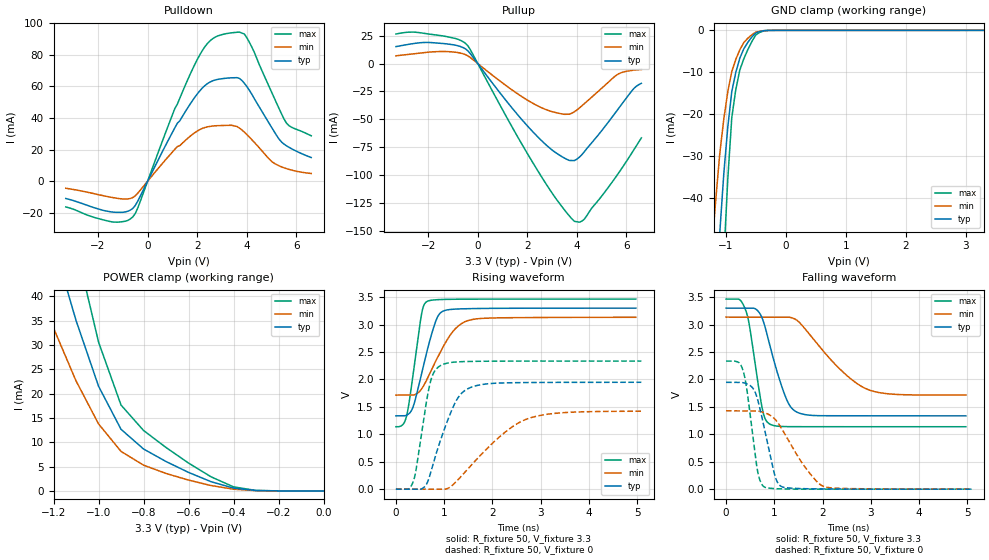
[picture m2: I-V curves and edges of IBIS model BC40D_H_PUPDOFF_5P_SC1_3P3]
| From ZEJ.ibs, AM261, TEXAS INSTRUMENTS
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[Model]   BC40D_H_PUPDOFF_5P_SC1_3P3
Model_type   I/O
Polarity   Non-Inverting
Enable   Active-Low
Vinl =  0.8V
Vinh =  2V
Cref =  15pF
Rref =  100.0000M
Vref =  0V
Vmeas =  1.65
C_comp   2.157014p   1.964007p   2.198404p
|[Input load] weak_pupdoff
|[Output drive] slow
|[supplytol] 5
|[temp] ind
[Model Spec]
Vinl   0.8V   0.8V   0.8V
Vinh   2V   2V   2V
[Temperature Range]   25   125   -40
[Voltage Range]   3.3   3.135   3.465
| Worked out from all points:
|   slope of the pulldown table from 0 to 0.495 V, typ, clamps not added: 31.8 ohm
|   slope of the pullup table from 0 to 0.495 V, typ, clamps not added: 33.8 ohm
|   GND clamp passes 1 mA (typ) near -0.53 V on its own axis
|   POWER clamp passes 1 mA (typ) near -0.43 V on its own axis
|   rising waveform, R_fixture 50, V_fixture 3.3: 20-80 % time 338ps typ, 517ps min, 220ps max; typ from 1.34 V to 3.3 V
|   rising waveform, R_fixture 50, V_fixture 0: 20-80 % time 469ps typ, 1.01ns min, 254ps max; typ from 0 V to 1.95 V
|   falling waveform, R_fixture 50, V_fixture 3.3: 20-80 % time 389ps typ, 896ps min, 241ps max; typ from 3.3 V to 1.34 V
|   falling waveform, R_fixture 50, V_fixture 0: 20-80 % time 295ps typ, 611ps min, 205ps max; typ from 1.95 V to 0 V
| Nom Voltages:
|   VDD=1.1, VDDS=3.3, VDDS18=1.8, ESD_BIASFET=0, VSS=0, VSSS=0
| Min Voltages:
|   VDD=1.045, VDDS=3.135, VDDS18=1.71, ESD_BIASFET=0, VSS=0, VSSS=0
| Max Voltages:
|   VDD=1.16, VDDS=3.465, VDDS18=1.89, ESD_BIASFET=0, VSS=0, VSSS=0
[POWER_clamp]
|   voltage   I(typ)   I(min)   I(max)
-3.3V     446.9mA    437.1mA    604mA
-1.267V   62.17mA    41.49mA    88.04mA
-1.233V   56.52mA    37.49mA    80.24mA
-1.133V   40.34mA    26.26mA    57.63mA
-1.067V   30.56mA    19.69mA    43.69mA
-1.033V   26.05mA    16.74mA    37.16mA
-1V       21.55mA    13.79mA    30.63mA
-900mV    12.68mA    8.13mA     17.66mA
-800mV    8.63mA     5.305mA    12.44mA
-600mV    3.813mA    2.231mA    5.735mA
-400mV    580.7uA    357.4uA    841.8uA
0V        4.589uA    2.331uA    8.159uA
[Pulldown]
|   voltage   I(typ)   I(min)   I(max)
-3.3V     -10.93mA   -4.474mA   -16.27mA
-1.4V     -19.53mA   -10.38mA   -25.83mA
-600mV    -17.23mA   -10.34mA   -22.61mA
1.2V      36.72mA    21.93mA    48.77mA
1.9V      53.02mA    30.66mA    73.76mA
2.4V      61.62mA    34.34mA    86.89mA
3V        64.86mA    35.24mA    92.76mA
3.6V      65.51mA    34.65mA    94.24mA
3.9V      62.01mA    31.1mA     93.16mA
5V        34.1mA     12.57mA    56.41mA
5.6V      22.42mA    7.958mA    36.79mA
6.6V      14.97mA    4.886mA    28.74mA
[Pullup]
|   voltage   I(typ)   I(min)   I(max)
-3.3V     15.12mA    6.907mA    26.36mA
-1.9V     18.73mA    10.27mA    26.12mA
-900mV    16.4mA     10.09mA    22.38mA
-400mV    11.39mA    6.888mA    15.9mA
1.3V      -37.44mA   -22.28mA   -53.31mA
2.4V      -65.08mA   -37.64mA   -95.03mA
3.2V      -80.46mA   -44.13mA   -122.1mA
3.9V      -86.71mA   -43.1mA    -141mA
4.3V      -78.82mA   -35.86mA   -139.1mA
5.6V      -42.54mA   -10.35mA   -100.4mA
6.3V      -22.29mA   -5.95mA    -77mA
6.6V      -17.71mA   -5.359mA   -66.44mA
[GND_clamp]
|   voltage   I(typ)   I(min)   I(max)
-3.3V     -787.2mA   -627.7mA   -1.235A
-1.233V   -85.66mA   -52.14mA   -138.8mA
-1.167V   -66.47mA   -40.37mA   -107.7mA
-1.1V     -48.25mA   -29.37mA   -77.98mA
-1.033V   -34.27mA   -21.19mA   -54.56mA
-966.7mV  -23.06mA   -14.66mA   -35.5mA
-900mV    -14.61mA   -9.789mA   -20.83mA
-833.3mV  -10.05mA   -6.934mA   -14.15mA
-700mV    -4.416mA   -2.931mA   -6.81mA
-500mV    -621.6uA   -443.6uA   -1.094mA
-300mV    -17.13uA   -24.35uA   -23.51uA
3.3V      4.589uA    5.188uA    6.318uA
[Ramp]
| variable   typ   min   max
dV/dt_f  1.1805377/0.38937067n 0.85643134/0.90272396n   1.398601/0.24138636n
dV/dt_r  1.1741843/0.47076543n 0.86234328/1.0203265n  1.4069047/0.25456543n
R_load = 50
[Rising Waveform]
R_fixture = 50
V_fixture = 3.3
V_fixture_min = 3.135
V_fixture_max = 3.465
|   time   V(typ)   V(min)   V(max)
0s        1.337V     1.714V     1.139V
142.6ps   1.337V     1.714V     1.175V
221.5ps   1.348V     1.714V     1.335V
358.3ps   1.505V     1.716V     2.104V
530.2ps   2.1V       1.824V     3.184V
644.1ps   2.514V     2.001V     3.42V
917.1ps   3.208V     2.493V     3.456V
1.21ns    3.281V     2.903V     3.461V
1.504ns   3.29V      3.075V     3.463V
4.974ns   3.3V       3.132V     3.465V
[Rising Waveform]
R_fixture = 50
V_fixture = 0
V_fixture_min = 0
V_fixture_max = 0
|   time   V(typ)   V(min)   V(max)
0s        0V         0V         0V
263.8ps   0V         0V         0V
361.7ps   0V         0V         145.6mV
579.9ps   30.57mV    0V         1.306V
709.1ps   267.1mV    0V         1.935V
934.7ps   919.7mV    0V         2.257V
1.28ns    1.657V     165.4mV    2.32V
1.635ns   1.879V     507.2mV    2.33V
2.798ns   1.944V     1.303V     2.335V
5.089ns   1.948V     1.421V     2.335V
[Falling Waveform]
R_fixture = 50
V_fixture = 3.3
V_fixture_min = 3.135
V_fixture_max = 3.465
|   time   V(typ)   V(min)   V(max)
0s        3.299V     3.135V     3.464V
275.8ps   3.299V     3.135V     3.457V
414.1ps   3.299V     3.135V     3.243V
750.7ps   3.114V     3.135V     1.47V
912.7ps   2.606V     3.135V     1.184V
1.258ns   1.631V     3.135V     1.14V
1.518ns   1.386V     3.04V      1.138V
2.338ns   1.338V     2.207V     1.138V
2.91ns    1.337V     1.827V     1.138V
4.974ns   1.336V     1.717V     1.138V
[Falling Waveform]
R_fixture = 50
V_fixture = 0
V_fixture_min = 0
V_fixture_max = 0
|   time   V(typ)   V(min)   V(max)
0s        1.947V     1.427V     2.334V
356.3ps   1.939V     1.427V     2.149V
438.5ps   1.917V     1.427V     1.774V
649.7ps   1.649V     1.424V     348.8mV
797.5ps   1.097V     1.393V     37.74mV
1.023ns   219mV      1.267V     8.661mV
1.177ns   38.17mV    1.069V     4.53mV
1.661ns   8.09mV     374mV      0V
2.048ns   4.365mV    43mV       0V
5.089ns   0V         2.137mV    0V
